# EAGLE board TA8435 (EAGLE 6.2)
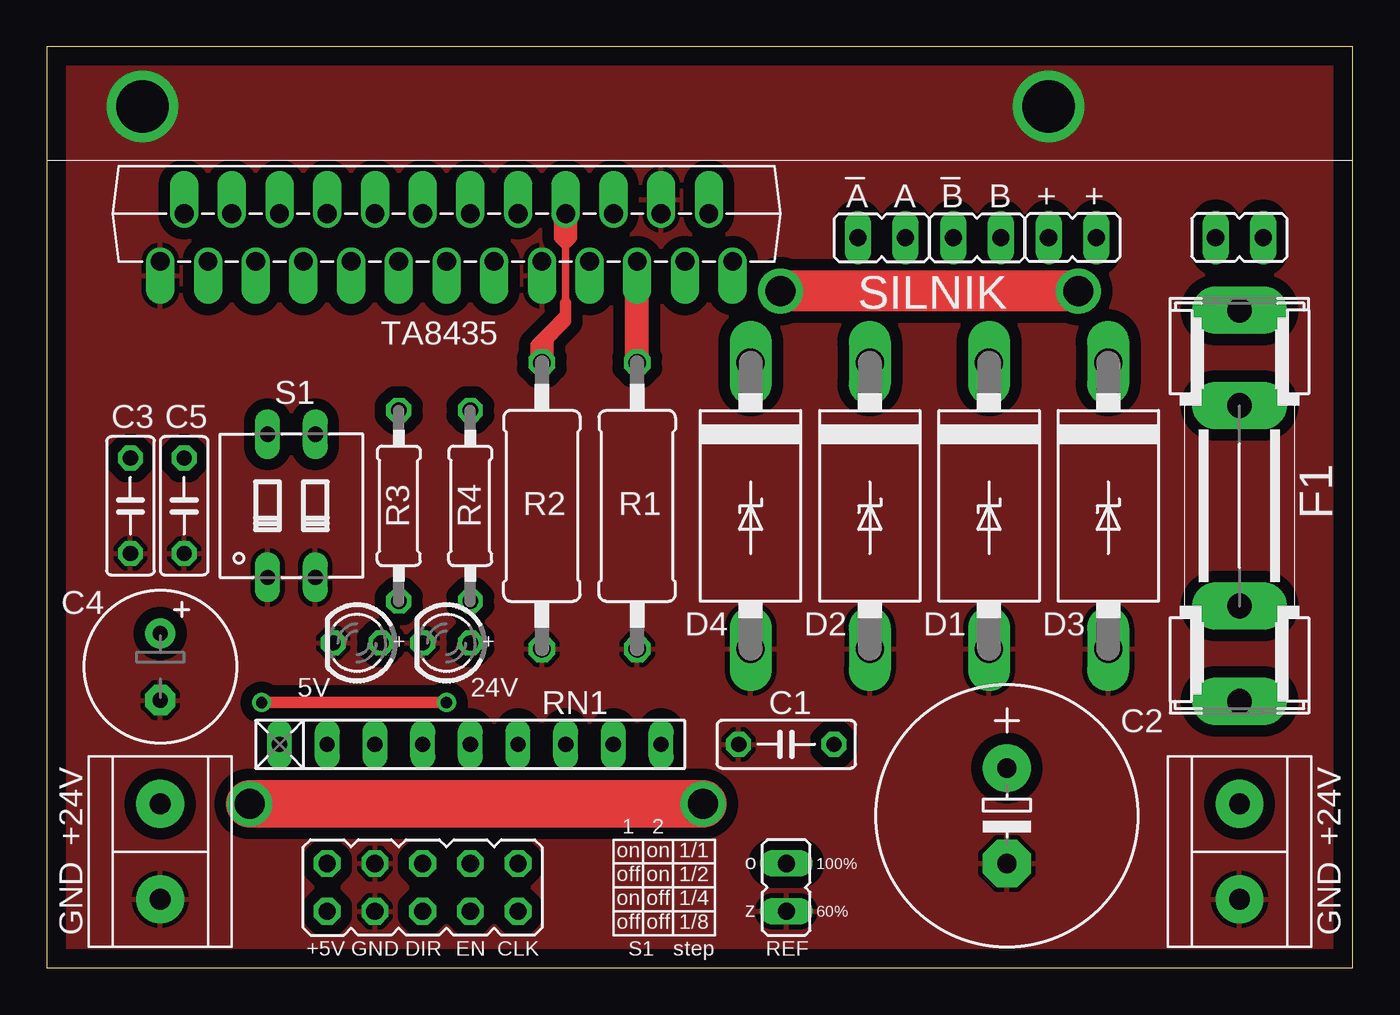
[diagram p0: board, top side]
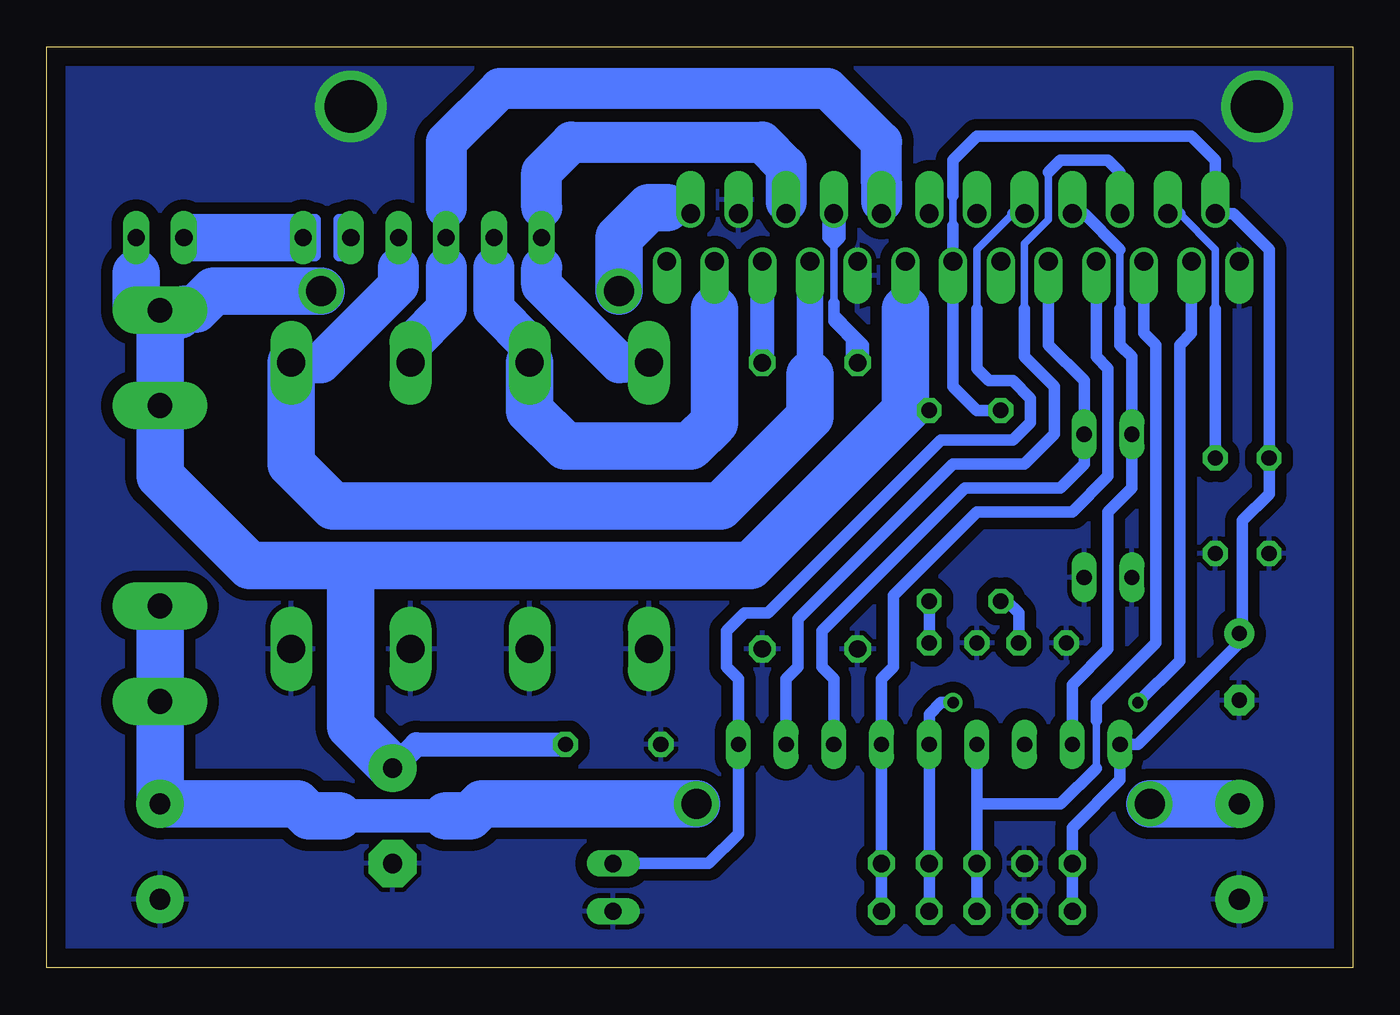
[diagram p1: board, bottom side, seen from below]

Size 69.52 x 49.04 mm. Coordinates in mm from the lower left corner, seen from the top.
Outline: 0,0 69.52,0 69.52,49.04 0,49.04 0,0
Copper layers (1*16): Top 0.035mm / dielectric 1.5mm / Bottom 0.035mm
Design rules: minimum track width 10mil, minimum drill 24mil, track to track 8mil, track to pad 8mil, pad to pad 8mil, via to via 8mil, smd to smd 8mil, copper to edge 40mil, drill to drill 8mil, minimum pad ring 10mil, minimum via ring 8mil, stop-mask expansion 4mil, vias tented up to drill 0mil, thermal gap 10mil

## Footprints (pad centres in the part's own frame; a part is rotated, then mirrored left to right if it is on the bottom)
C050-025X075 = drill 0.813 octagon: 1 -2.54,0; 2 2.54,0
E5-13 = drill 1.016 pad 2.54: + -2.54,0 | drill 1.016 pad 2.54 octagon: - 2.54,0
E3,5-8 = drill 0.813 pad 1.6: + -1.778,0 | drill 0.813 pad 1.6 octagon: - 1.778,0
C4111-15 = drill 1.499 long: A 7.62,0; C -7.62,0
SHK20L = drill 1.321 pad 2.54 long: 1A -10.414,0; 1B -5.334,0; 2A 10.414,0; 2B 5.334,0
JP1 = drill 0.914 long: 1 0,-1.27; 2 0,1.27
JP5Q = drill 0.914 octagon: 1 -5.08,-1.27; 2 -5.08,1.27; 3 -2.54,-1.27; 4 -2.54,1.27; 5 0,-1.27; 6 0,1.27; 7 2.54,-1.27; 8 2.54,1.27; 9 5.08,-1.27; 10 5.08,1.27
LED3MM = drill 0.813 octagon: A -1.27,0; K 1.27,0
0411/15 = drill 0.914 octagon: 1 -7.62,0; 2 7.62,0
0207/10 = drill 0.813 pad 1.27 octagon: 1 -5.08,0; 2 5.08,0
RN-9 = drill 0.813 long: 1 -10.16,0; 2 -7.62,0; 3 -5.08,0; 4 -2.54,0; 5 0,0; 6 2.54,0; 7 5.08,0; 8 7.62,0; 9 10.16,0
DIP02YL = drill 0.813 long: 1 -1.27,-3.81; 2 1.27,-3.81; 3 1.27,3.81; 4 -1.27,3.81
TA8435 = drill 1 offset: P$1 -15.24,-1.27; P$2 -13.97,1.27; P$3 -12.7,-1.27; P$4 -11.43,1.27; P$5 -10.16,-1.27; P$6 -8.89,1.27; P$7 -7.62,-1.27; P$8 -6.35,1.27; P$9 -5.08,-1.27; P$10 -3.81,1.27; P$11 -2.54,-1.27; P$12 -1.27,1.27; P$13 0,-1.27; P$14 1.27,1.27; P$15 2.54,-1.27; P$16 3.81,1.27; P$17 5.08,-1.27; P$18 6.35,1.27; P$19 7.62,-1.27; P$20 8.89,1.27; P$21 10.16,-1.27; P$22 11.43,1.27; P$23 12.7,-1.27; P$24 13.97,1.27; P$25 15.24,-1.27
ARK2 = drill 1.1 pad 2.54: P$1 -2.54,0; P$2 2.54,0

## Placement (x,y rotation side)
C1  [C050-025X075]  39.37,11.91 180 top
C2  [E5-13]  51.12,8.1 270 top
C3  [C050-025X075]  4.45,24.61 270 top
C4  [E3,5-8]  6.03,16.03 270 top
C5  [C050-025X075]  7.3,24.61 270 top
D1  1N5908  [C4111-15]  50.16,24.61 270 top
D2  1N5908  [C4111-15]  43.82,24.61 270 top
D3  1N5908  [C4111-15]  56.52,24.61 270 top
D4  1N5908  [C4111-15]  37.47,24.61 270 top
F1  [SHK20L]  63.5,24.61 90 top
JP1  [JP1]  44.45,38.89 90 top
JP2  [JP1]  54.61,38.89 270 top
JP3  [JP1]  49.53,38.89 90 top
JP4  [JP1]  39.37,4.29 180 top
JP5  [JP1]  63.5,38.89 270 top
JP6  [JP5Q]  20,4.29 0 top
LED1  [LED3MM]  16.51,17.3 180 top
LED2  [LED3MM]  21.27,17.3 180 top
R1  [0411/15]  31.43,24.61 90 top
R2  [0411/15]  26.35,24.61 270 top
R3  [0207/10]  18.73,24.61 270 top
R4  [0207/10]  22.54,24.61 270 top
RN1  [RN-9]  22.54,11.91 0 top
S1  [DIP02YL]  13.02,24.61 0 top
U$1  TA8435  [TA8435]  21.27,38.89 0 top
U$2  ARK2  [ARK2]  63.5,6.19 270 top
U$4  ARK2  [ARK2]  6.03,6.19 90 top

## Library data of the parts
C1-C5 R1-R4 = rcl
D1-D4 = diode
F1 = fuse
JP1-JP6 = jumper
LED1 LED2 = led
RN1 = resistor-net
S1 = switch-dil
U$1 = ta8435
U$2 U$4 = !ark2m

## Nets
GND: C1.2 C2.- C3.2 C4.- C5.2 D1.A D2.A D3.A D4.A JP4.2 JP6.3 JP6.4 LED1.K LED2.K R1.1 R2.2 S1.1 S1.2 U$1.P$1 U$1.P$17 U$1.P$22 U$2.P$2 U$4.P$1
N$1: D2.C JP1.1 U$1.P$23
N$2: D4.C JP1.2 U$1.P$20
N$3: D3.C JP3.1 U$1.P$19
N$4: D1.C JP3.2 U$1.P$16
N$5: R1.2 U$1.P$21
N$7: F1.1A U$2.P$1 U$4.P$2
N$8: C3.1 C4.+ JP6.1 JP6.2 R3.1 RN1.1 U$1.P$2 U$1.P$13
N$9: JP4.1 RN1.9 U$1.P$10
N$10: C1.1 C2.+ F1.2A R4.1 U$1.P$15 U$1.P$24
N$11: JP6.7 JP6.8 RN1.5 U$1.P$3
N$12: RN1.8 U$1.P$6
N$13: JP6.9 JP6.10 RN1.6 U$1.P$7
N$14: RN1.2 S1.4 U$1.P$8
N$15: RN1.7 S1.3 U$1.P$9
N$16: C5.1 U$1.P$4
N$17: JP6.5 JP6.6 RN1.4 U$1.P$5
N$18: LED2.A R4.2
N$19: JP2.2 JP5.1
N$20: LED1.A R3.2
N$23: R2.1 U$1.P$18

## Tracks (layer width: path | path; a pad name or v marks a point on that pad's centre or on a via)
GND  (via drill 2.8)
  other vias: 5.08,45.88 53.34,45.88 5.08,45.88 53.34,45.88 5.08,45.88 53.34,45.88
  pour Top (isolate 0.61): 0,49.37 0,-0.16 69.85,-0.48 69.85,49.05
  pour Bottom (isolate 0.61): 0.16,49.21 -0.16,-0.32 69.85,-0.16 70.17,49.37
N$1
  Bottom 0.61: 33.97,35.08 U$1.P$23 | 45.72,37.31 JP1.1
  Bottom 2.184: D2.C 43.82,33.18 45.72,35.08 45.72,37.31
  Bottom 2.54: D2.C 43.82,29.69 41.91,27.78 35.24,27.78 33.97,29.05 33.97,35.08
N$2
  Bottom 0.61: 30.16,42.7 U$1.P$20 | 43.18,37.31 JP1.2 43.18,40.48
  Bottom 2.184: 30.16,40.8 30.16,42.7 31.43,43.97 41.59,43.97 43.18,42.39 43.18,40.48 | D4.C 39.05,32.23 43.18,36.35 43.18,37.31
N$3
  Bottom 0.61: 50.8,37.31 JP3.1
  Bottom 1.422: 28.89,31.59 U$1.P$19
  Bottom 2.184: D3.C 54.93,32.23 50.8,36.35 50.8,37.31
  Bottom 2.54: D3.C 56.52,26.83 54.29,24.61 33.66,24.61 28.89,29.37 28.89,31.59
N$4
  Bottom 0.61: U$1.P$16 25.08,41.75 | 48.26,37.31 JP3.2 48.26,40.48
  Bottom 2.184: 25.08,40.8 25.08,41.75 25.08,43.97 27.94,46.83 45.4,46.83 48.26,43.97 48.26,40.48 | D1.C 50.16,33.18 48.26,35.08 48.26,37.31
N$5
  Top 0.61: R1.2 U$1.P$21
  Top 0.813: R1.2 U$1.P$21
  Top 1.016: R1.2 U$1.P$21
  Top 1.27: R1.2 U$1.P$21
  Bottom 0.61: R1.2 U$1.P$21
  Bottom 0.813: R1.2 U$1.P$21
  Bottom 1.27: R1.2 U$1.P$21
N$6
  Bottom 0.61: 53.34,39.85 53.98,39.85 53.98,37.94 53.34,37.94 53.34,39.85 | 53.34,39.85 53.66,39.85 53.66,38.26
N$7  (via drill 1.6)
  Top 2.54: v10.8,8.73 v34.93,8.73
  Bottom 1.778: 48.26,8.1 53.98,8.1
  Bottom 2.54: v34.93,8.73 46.35,8.73 46.99,8.1 48.26,8.1 | 53.98,8.1 55.56,8.1 56.2,8.73 U$2.P$1 F1.1A 63.5,19.21 | U$4.P$2 v10.8,8.73
N$8
  Bottom 0.406: 21.27,41.12 21.27,39.53
  Bottom 0.61: R3.1 20,29.69 21.27,30.96 U$1.P$13 21.27,39.53 | 21.27,41.12 21.27,43.02 20,44.29 8.57,44.29 7.3,43.02 U$1.P$2 6.35,40.16 4.44,38.26 C3.1 4.44,25.24 5.87,23.81 5.87,18.42 6.16,18.13 C4.+ 6.03,17.3 11.43,11.91 RN1.1 12.38,10 14.92,7.46 JP6.2 JP6.1
N$9
  Bottom 0.406: 20,35.08 20,38.26 18.1,40.16
  Bottom 0.61: 18.1,40.16 U$1.P$10 | 20,33.5 20,33.18 | 20,33.5 20,31.91 19.37,31.27 18.1,31.27 17.15,30.32 17.15,29.05 18.1,28.1 21.91,28.1 31.12,18.89 32.38,18.89 33.34,17.94 33.34,16.03 32.7,15.4 RN1.9 32.7,7.14 34.29,5.56 JP4.1 | 20,33.5 20,35.08
N$10  (via drill 1.6)
  Top 0.61: v54.93,36.04 v39.05,36.04
  Top 2.184: v54.93,36.04 v39.05,36.04
  Bottom 0.61: 62.17,35.08 61.6,35.08 | 55.24,21.43 53.34,21.11 | 35.56,40.48 U$1.P$24 | 23.81,35.08 U$1.P$15 | R4.1 23.81,29.69
  Bottom 1.27: 53.34,21.11 53.34,12.86 | C1.1 49.85,11.91 C2.+
  Bottom 1.93: 36.51,40.48 35.56,40.48
  Bottom 2.54: v54.93,36.04 60.64,36.04 61.6,35.08 | 23.81,35.08 23.81,29.69 32.07,21.43 53.34,21.43 | 53.34,21.43 55.24,21.43 58.74,21.43 63.5,26.19 63.5,34.77 | 36.51,40.48 37.47,40.48 39.05,38.89 v39.05,36.04 | 64.77,35.08 64.45,35.08 | 64.77,35.08 64.77,36.99 | 63.5,34.77 F1.2A 64.71,35.02 64.77,35.08 | 63.5,34.77 62.48,34.77 62.17,35.08 | 53.34,21.43 53.34,21.11 | 53.34,21.43 53.34,12.86 C2.+
N$11  (via drill 0.6)
  Top 0.61: v11.43,14.13 v21.27,14.13
  Bottom 0.61: v11.43,14.13 9.21,16.35 9.21,33.18 8.57,33.81 U$1.P$3 | v21.27,14.13 21.91,14.13 22.54,13.49 RN1.5 JP6.8 JP6.7
N$12
  Bottom 0.406: 16.19,42.39 16.19,39.85 17.46,38.58 17.46,35.08
  Bottom 0.61: RN1.8 30.16,15.4 29.53,16.03 29.53,18.57 21.27,26.83 17.46,26.83 15.87,28.42 15.87,30.96 17.46,32.54 17.46,35.08 | U$1.P$6 12.38,42.39 13.02,43.02 15.56,43.02 16.19,42.39
N$13
  Bottom 0.61: U$1.P$7 13.65,32.54 13.02,31.91 13.02,26.19 14.92,24.29 20,24.29 24.45,19.84 24.45,16.03 25.08,15.4 RN1.6 | RN1.6 25.08,11.59 | JP6.9 JP6.10 RN1.6
N$14
  Bottom 0.406: 12.38,35.08 12.38,38.26
  Bottom 0.61: U$1.P$8 14.29,40.16 12.38,38.26 | RN1.2 14.92,15.08 13.02,16.99 13.02,24.29 11.75,25.56 S1.4 11.75,32.54 12.38,33.18 12.38,35.08
N$15
  Bottom 0.61: U$1.P$9 16.19,33.18 14.29,31.27 S1.3 14.29,26.83 15.56,25.56 20.64,25.56 28.26,17.94 28.26,16.03 27.62,15.4 RN1.7
N$16
  Bottom 0.406: 7.3,35.08 7.3,38.26 9.21,40.16
  Bottom 0.61: 9.21,40.16 U$1.P$4 | C5.1 7.3,35.08
N$17
  Bottom 0.406: 13.65,10.64 13.65,13.18
  Bottom 0.61: 13.65,10.64 15.56,8.73 20,8.73 | U$1.P$5 11.11,33.81 10.48,33.18 10.48,17.3 13.65,14.13 13.65,13.18 | JP6.5 JP6.6 20,8.73 | 20,8.73 RN1.4
N$18
  Bottom 0.61: LED2.A R4.2
N$19
  Bottom 0.61: JP2.2 56.52,38.89 | 61.6,38.89 JP5.1
  Bottom 2.54: 56.52,38.89 57.15,38.89 61.6,38.89
N$20
  Bottom 0.61: LED1.A 17.78,18.89 18.41,19.53 R3.2
N$21
  Bottom 0.61: 55.88,39.85 55.24,39.85 55.24,37.94 55.88,37.94 55.88,39.85 | 55.88,39.85 55.56,39.85 55.56,38.26
N$22
  Bottom 0.61: 7.3,27.46 7.3,34.13
N$23
  Top 0.406: 27.62,35.4 27.62,38.58
  Top 0.61: 27.62,38.58 U$1.P$18 | 27.62,34.77 27.62,35.4 | 26.67,33.81 26.35,33.5 R2.1 | 27.62,38.58 27.3,38.89 27.3,40.16 27.94,40.16 27.94,38.89 27.62,38.58 | R2.1 26.04,32.23 26.04,33.18 | 26.67,33.81 26.04,33.18 | 26.67,33.81 27.62,34.77 | 26.67,33.81 26.67,32.23 R2.1 | 26.04,33.18 26.35,33.18 27.62,34.45 27.62,34.77
  Bottom 0.406: 27.62,35.4 27.62,38.58
  Bottom 0.61: 27.62,34.77 27.62,35.4 | 26.67,33.81 26.35,33.5 26.35,33.18 | 26.67,33.81 27.62,34.77 | R2.1 26.35,33.18 | 27.62,38.58 U$1.P$18 | 27.62,38.58 27.3,38.89 27.3,40.16 27.94,40.16 27.94,38.89 27.62,38.58 | 26.67,33.81 26.67,32.23 R2.1 | 26.67,33.81 26.04,33.18 26.04,32.23 R2.1 | 27.62,34.77 27.62,34.45 26.35,33.18

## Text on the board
tPlace: A | A | B | B | + | + | SILNIK | + | + | 5V | 24V | 1 | 2 | +24V | on | on | 1/1 | +24V | o | 100% | off | on | 1/2 | on | off | 1/4 | z | 60% | GND | off | off | 1/8 | GND | +5V | GND | DIR | EN | CLK | S1 | step | REF
tStop: Piotr Witczak
bStop: Piotr Witczak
